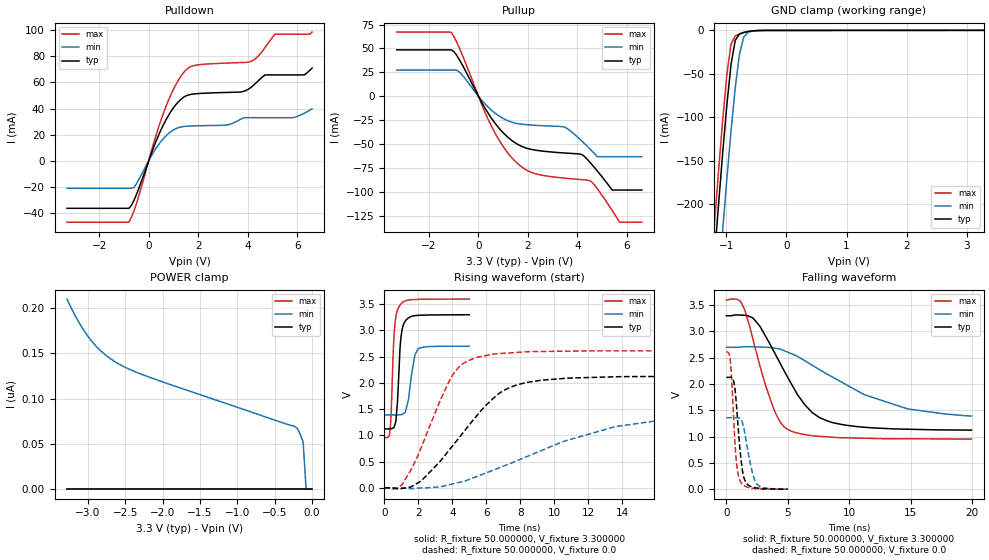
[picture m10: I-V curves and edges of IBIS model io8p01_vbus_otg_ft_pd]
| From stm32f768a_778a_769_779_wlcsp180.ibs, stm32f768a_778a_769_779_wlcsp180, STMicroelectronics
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|   Model io8p01_vbus_otg_ft_pd
[Model]  io8p01_vbus_otg_ft_pd
Model_type I/O
Polarity   Non-Inverting
Enable   Active-Low
Vinl =   0.990000V
Vinh =   2.310000V
Vmeas =  1.650000V
Cref =   50.000000pF
Rref =   100.000000M
Vref =   0.0V
C_comp   3.304800pF   3.199300pF   3.429300pF
[Temperature Range]   25.000000   0.125000k   -40.000000
[Pullup Reference]   3.300000V   2.700000V   3.600000V
[Pulldown Reference]   0.0V   0.0V   0.0V
[POWER Clamp Reference]   3.300000V   2.700000V   3.600000V
[GND Clamp Reference]   0.0V   0.0V   0.0V
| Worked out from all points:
|   slope of the pulldown table from 0 to 0.495 V, typ, clamps not added: 20.9 ohm
|   slope of the pullup table from 0 to 0.495 V, typ, clamps not added: 22.6 ohm
|   GND clamp passes 1 mA (typ) near -0.61 V on its own axis
|   rising waveform, R_fixture 50.000000, V_fixture 3.300000: 20-80 % time 225ps typ, 352ps min, 207ps max; typ from 1.12 V to 3.3 V
|   rising waveform, R_fixture 50.000000, V_fixture 0.0: 20-80 % time 3.35ns typ, 6.83ns min, 2.07ns max; typ from 0 V to 2.13 V
|   falling waveform, R_fixture 50.000000, V_fixture 3.300000: 20-80 % time 3.28ns typ, 6.7ns min, 2.02ns max; typ from 3.3 V to 1.12 V
|   falling waveform, R_fixture 50.000000, V_fixture 0.0: 20-80 % time 480ps typ, 678ps min, 386ps max; typ from 2.13 V to 0 V
[Pulldown]
|Voltage   I(typ)   I(min)   I(max)
-3.3V     -36.41mA   -21.08mA   -47.03mA
-800mV    -36.41mA   -21.08mA   -47.03mA
-600mV    -30.48mA   -20.53mA   -38.65mA
700mV     31.4mA     19.11mA    41.71mA
1.2V      45.15mA    25.37mA    61.75mA
1.6V      50.35mA    26.5mA     71.06mA
3.1V      52.27mA    27.26mA    74.75mA
4.1V      55.7mA     32.99mA    75.8mA
4.7V      65.72mA    32.99mA    86.69mA
5.1V      65.72mA    32.99mA    96.9mA
6.3V      65.87mA    36.5mA     96.9mA
6.6V      70.93mA    39.71mA    98.5mA
[Pullup]
|Voltage   I(typ)   I(min)   I(max)
-3.3V     48.54mA    27.43mA    67.18mA
-1.1V     48.54mA    27.43mA    66.9mA
-700mV    35.13mA    23.47mA    46.35mA
500mV     -22.07mA   -14mA      -30.03mA
1.5V      -49.1mA    -28.3mA    -68.56mA
2.2V      -56.04mA   -30.32mA   -80.35mA
3.5V      -59.53mA   -32.66mA   -85.92mA
4.5V      -69.06mA   -55.13mA   -88.4mA
4.8V      -78.22mA   -63.4mA    -96.84mA
5.4V      -98.3mA    -63.4mA    -119.6mA
5.7V      -98.3mA    -63.4mA    -132mA
6.6V      -98.3mA    -63.4mA    -132mA
[GND_clamp]
|Voltage   I(typ)   I(min)   I(max)
-3.3V     -2.319A    -2.398A    -2.292A
-1.2V     -265.6mA   -356.2mA   -227.3mA
-1.13V    -202.8mA   -293mA     -164.3mA
-1.06V    -142.3mA   -231.2mA   -104.3mA
-990mV    -86.15mA   -171.7mA   -51.01mA
-920mV    -39.05mA   -115.6mA   -15.73mA
-850mV    -11.41mA   -65.74mA   -6.38mA
-780mV    -4.058mA   -27.6mA    -4.167mA
-710mV    -2.296mA   -7.89mA    -2.605mA
-640mV    -1.302mA   -2.283mA   -1.381mA
-570mV    -629.1uA   -918.9uA   -580.8uA
3.28V     81.28uA    57.87uA    93.98uA
[POWER_clamp]
|Voltage   I(typ)   I(min)   I(max)
-3.28V    0A         210.1nA    0A
-3.12V    0A         184.2nA    0A
-2.96V    0A         164.6nA    0A
-2.8V     0A         150.7nA    0A
-2.6V     0A         139nA      0A
-2.16V    0A         123.2nA    0A
-240mV    0A         69.7nA     0A
-200mV    0A         67.32nA    0A
-160mV    0A         60.72nA    0A
-120mV    0A         52.23nA    0A
-80mV     0A         0A         0A
0V        0A         0A         0A
[Ramp]
| variable   typ   min   max
dV/dt_r  1.27908/3.35593n   0.79842/6.85470n   1.56666/2.07175n
dV/dt_f  1.30224/3.28286n   0.73974/6.61202n   1.58738/2.01513n
R_load = 50.000000
[Rising Waveform]
R_fixture= 50.000000
V_fixture= 3.300000
V_fixture_min= 2.700000
V_fixture_max= 3.600000
|time   V(typ)   V(min)   V(max)
0s        1.123V     1.391V     954mV
300.3ps   1.125V     1.391V     1.026V
370.4ps   1.127V     1.391V     1.284V
580.6ps   1.171V     1.391V     2.988V
670.7ps   1.279V     1.39V      3.258V
850.9ps   2.212V     1.391V     3.45V
930.9ps   2.735V     1.392V     3.488V
1.101ns   3.099V     1.414V     3.543V
1.992ns   3.287V     2.657V     3.592V
4.985ns   3.299V     2.699V     3.598V
[Rising Waveform]
R_fixture= 50.000000
V_fixture= 0.0
V_fixture_min= 0.0
V_fixture_max= 0.0
|time   V(typ)   V(min)   V(max)
0s        358.2uV    202.6uV    672.5uV
1.081ns   -9.469mV   -1.93mV    83.55mV
2.162ns   131.4mV    -2.589mV   771.7mV
3.804ns   719.2mV    59.2mV     2.03V
4.284ns   913.5mV    95.95mV    2.268V
4.885ns   1.158V     147.4mV    2.419V
6.727ns   1.796V     379.3mV    2.558V
8.448ns   2.012V     605mV      2.595V
13.61ns   2.116V     1.169V     2.61V
19.94ns   2.127V     1.357V     2.611V
[Falling Waveform]
R_fixture= 50.000000
V_fixture= 3.300000
V_fixture_min= 2.700000
V_fixture_max= 3.600000
|time   V(typ)   V(min)   V(max)
0s        3.299V     2.699V     3.598V
880.9ps   3.313V     2.699V     3.611V
1.441ns   3.308V     2.709V     3.437V
2.202ns   3.245V     2.707V     2.81V
3.644ns   2.716V     2.691V     1.663V
5.045ns   2.103V     2.6V       1.13V
6.967ns   1.46V      2.359V     1.017V
8.609ns   1.268V     2.135V     988.7mV
14.73ns   1.141V     1.527V     958.3mV
19.94ns   1.123V     1.391V     954mV
[Falling Waveform]
R_fixture= 50.000000
V_fixture= 0.0
V_fixture_min= 0.0
V_fixture_max= 0.0
|time   V(typ)   V(min)   V(max)
0s        2.127V     1.357V     2.611V
300.3ps   2.129V     1.357V     2.476V
460.5ps   2.117V     1.357V     1.94V
620.6ps   2.018V     1.357V     1.196V
810.8ps   1.614V     1.359V     516.1mV
1.111ns   734mV      1.343V     160.1mV
1.491ns   173.4mV    1.071V     59.83mV
2.142ns   38.16mV    283.5mV    15.34mV
2.452ns   23.01mV    107.1mV    10.12mV
4.985ns   358.2uV    202.6uV    672.5uV
